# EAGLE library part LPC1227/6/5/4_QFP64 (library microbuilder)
LPC1227/6/5/4 - 32-bit ARM Cortex-M0 microcontroller - LQFP64 Package Low-Power ARM Cortex-M0 up to 33MHz Up to 8KB SRAM / 128KB Flash Digital Peripherals: Micro DMA Controller, CRC Engine, 2xUART, SSP/SPI, I2C, 2x 32-bit Timers, 2x16-bit Timers Analog Periherals: 8-Channel 10-bit ADC, 2 Analog Comparators
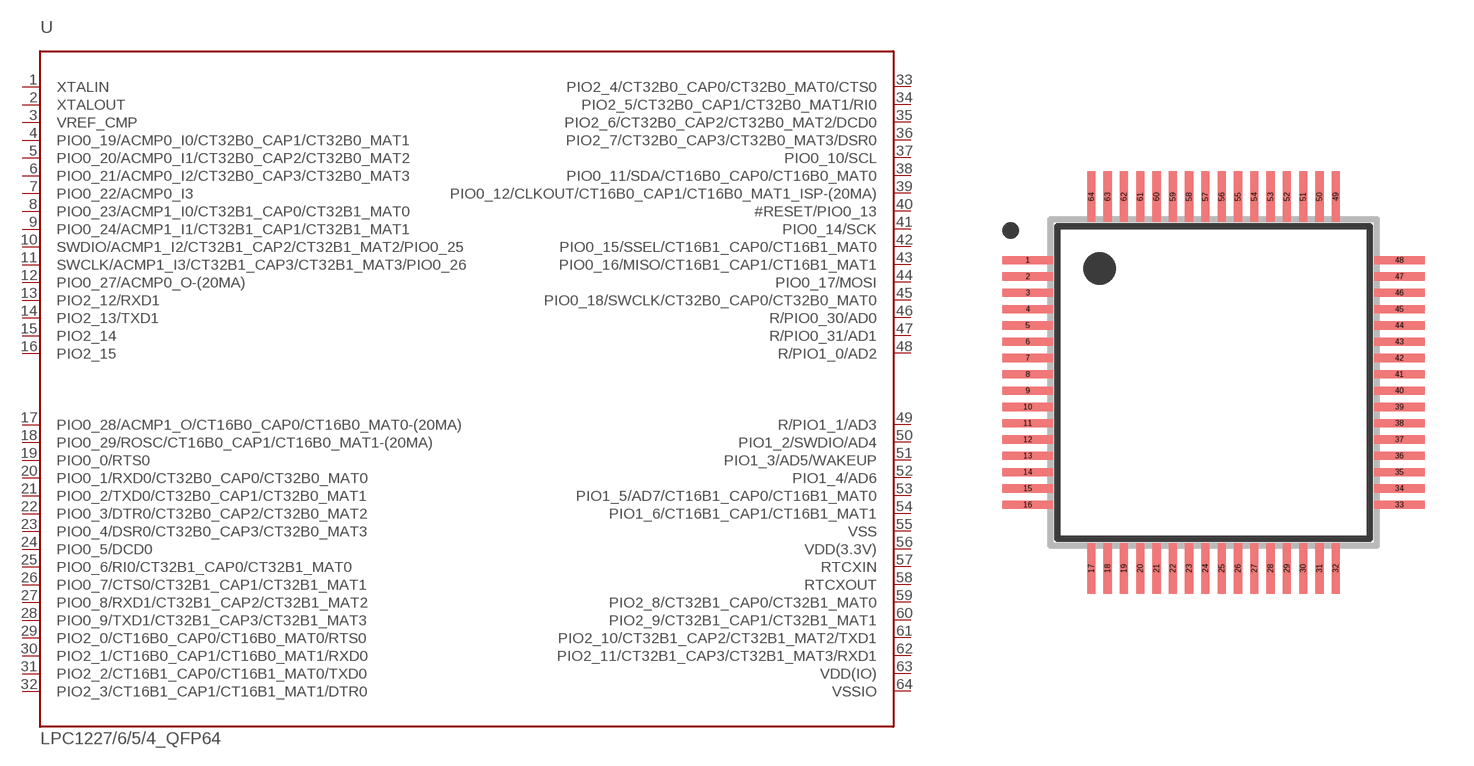
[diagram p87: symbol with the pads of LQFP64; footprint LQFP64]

Designator prefix U

## LPC1227/6/5/4_QFP64  [LQFP64]
1  XTALIN
2  XTALOUT
3  VREF_CMP
4  PIO0_19/ACMP0_I0/CT32B0_CAP1/CT32B0_MAT1
5  PIO0_20/ACMP0_I1/CT32B0_CAP2/CT32B0_MAT2
6  PIO0_21/ACMP0_I2/CT32B0_CAP3/CT32B0_MAT3
7  PIO0_22/ACMP0_I3
8  PIO0_23/ACMP1_I0/CT32B1_CAP0/CT32B1_MAT0
9  PIO0_24/ACMP1_I1/CT32B1_CAP1/CT32B1_MAT1
10  SWDIO/ACMP1_I2/CT32B1_CAP2/CT32B1_MAT2/PIO0_25
11  SWCLK/ACMP1_I3/CT32B1_CAP3/CT32B1_MAT3/PIO0_26
12  PIO0_27/ACMP0_O-(20MA)
13  PIO2_12/RXD1
14  PIO2_13/TXD1
15  PIO2_14
16  PIO2_15
17  PIO0_28/ACMP1_O/CT16B0_CAP0/CT16B0_MAT0-(20MA)
18  PIO0_29/ROSC/CT16B0_CAP1/CT16B0_MAT1-(20MA)
19  PIO0_0/RTS0
20  PIO0_1/RXD0/CT32B0_CAP0/CT32B0_MAT0
21  PIO0_2/TXD0/CT32B0_CAP1/CT32B0_MAT1
22  PIO0_3/DTR0/CT32B0_CAP2/CT32B0_MAT2
23  PIO0_4/DSR0/CT32B0_CAP3/CT32B0_MAT3
24  PIO0_5/DCD0
25  PIO0_6/RI0/CT32B1_CAP0/CT32B1_MAT0
26  PIO0_7/CTS0/CT32B1_CAP1/CT32B1_MAT1
27  PIO0_8/RXD1/CT32B1_CAP2/CT32B1_MAT2
28  PIO0_9/TXD1/CT32B1_CAP3/CT32B1_MAT3
29  PIO2_0/CT16B0_CAP0/CT16B0_MAT0/RTS0
30  PIO2_1/CT16B0_CAP1/CT16B0_MAT1/RXD0
31  PIO2_2/CT16B1_CAP0/CT16B1_MAT0/TXD0
32  PIO2_3/CT16B1_CAP1/CT16B1_MAT1/DTR0
33  PIO2_4/CT32B0_CAP0/CT32B0_MAT0/CTS0
34  PIO2_5/CT32B0_CAP1/CT32B0_MAT1/RI0
35  PIO2_6/CT32B0_CAP2/CT32B0_MAT2/DCD0
36  PIO2_7/CT32B0_CAP3/CT32B0_MAT3/DSR0
37  PIO0_10/SCL
38  PIO0_11/SDA/CT16B0_CAP0/CT16B0_MAT0
39  PIO0_12/CLKOUT/CT16B0_CAP1/CT16B0_MAT1_ISP-(20MA)
40  #RESET/PIO0_13
41  PIO0_14/SCK
42  PIO0_15/SSEL/CT16B1_CAP0/CT16B1_MAT0
43  PIO0_16/MISO/CT16B1_CAP1/CT16B1_MAT1
44  PIO0_17/MOSI
45  PIO0_18/SWCLK/CT32B0_CAP0/CT32B0_MAT0
46  R/PIO0_30/AD0
47  R/PIO0_31/AD1
48  R/PIO1_0/AD2
49  R/PIO1_1/AD3
50  PIO1_2/SWDIO/AD4
51  PIO1_3/AD5/WAKEUP
52  PIO1_4/AD6
53  PIO1_5/AD7/CT16B1_CAP0/CT16B1_MAT0
54  PIO1_6/CT16B1_CAP1/CT16B1_MAT1
55  VSS
56  VDD(3.3V)
57  RTCXIN
58  RTCXOUT
59  PIO2_8/CT32B1_CAP0/CT32B1_MAT0
60  PIO2_9/CT32B1_CAP1/CT32B1_MAT1
61  PIO2_10/CT32B1_CAP2/CT32B1_MAT2/TXD1
62  PIO2_11/CT32B1_CAP3/CT32B1_MAT3/RXD1
63  VDD(IO)
64  VSSIO

## Footprint LQFP64 (pad centres in mm)
smd 1.55 x 0.25: 1 -5.7,3.75; 2 -5.7,3.25; 3 -5.7,2.75; 4 -5.7,2.25; 5 -5.7,1.75; 6 -5.7,1.25; 7 -5.7,0.75; 8 -5.7,0.25; 9 -5.7,-0.25; 10 -5.7,-0.75; 11 -5.7,-1.25; 12 -5.7,-1.75; 13 -5.7,-2.25; 14 -5.7,-2.75; 15 -5.7,-3.25; 16 -5.7,-3.75; 33 5.7,-3.75; 34 5.7,-3.25; 35 5.7,-2.75; 36 5.7,-2.25; 37 5.7,-1.75; 38 5.7,-1.25; 39 5.7,-0.75; 40 5.7,-0.25; 41 5.7,0.25; 42 5.7,0.75; 43 5.7,1.25; 44 5.7,1.75; 45 5.7,2.25; 46 5.7,2.75; 47 5.7,3.25; 48 5.7,3.75
smd 0.25 x 1.55: 17 -3.75,-5.7; 18 -3.25,-5.7; 19 -2.75,-5.7; 20 -2.25,-5.7; 21 -1.75,-5.7; 22 -1.25,-5.7; 23 -0.75,-5.7; 24 -0.25,-5.7; 25 0.25,-5.7; 26 0.75,-5.7; 27 1.25,-5.7; 28 1.75,-5.7; 29 2.25,-5.7; 30 2.75,-5.7; 31 3.25,-5.7; 32 3.75,-5.7; 49 3.75,5.7; 50 3.25,5.7; 51 2.75,5.7; 52 2.25,5.7; 53 1.75,5.7; 54 1.25,5.7; 55 0.75,5.7; 56 0.25,5.7; 57 -0.25,5.7; 58 -0.75,5.7; 59 -1.25,5.7; 60 -1.75,5.7; 61 -2.25,5.7; 62 -2.75,5.7; 63 -3.25,5.7; 64 -3.75,5.7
